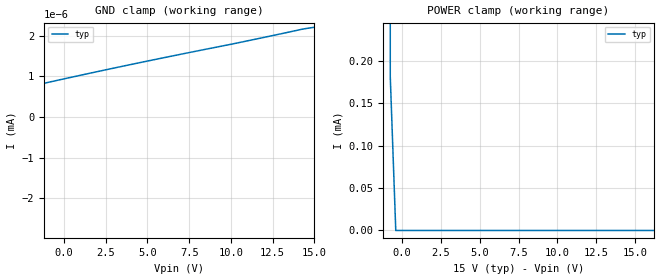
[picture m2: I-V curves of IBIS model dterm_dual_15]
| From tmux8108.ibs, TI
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| dterm_dual_15
[Model]   dterm_dual_15
Model_type   Terminator
|   typ   min   max
C_comp   1.008417e-11   NA   NA
[Voltage Range]   15   NA   NA
[Temperature Range]   27   NA   NA
[Power Clamp Reference]   15   NA   NA
[GND Clamp Reference]   0   NA   NA
[GND Clamp]
|   Voltage   I(typ)   I(min)   I(max)
-20V      -4.512A    NA         NA
-15.4V    -86.77nA   NA         NA
-15.05V   -296.1pA   NA         NA
-11.87V   -106.3pA   NA         NA
-9.394V   81.01pA    NA         NA
2.626V    1.175nA    NA         NA
15V       2.212nA    NA         NA
[POWER Clamp]
|   Voltage   I(typ)   I(min)   I(max)
-5V       1.488A     NA         NA
-1.111V   52.26mA    NA         NA
-757.6mV  181uA      NA         NA
-404mV    2.957nA    NA         NA
30V       -293pA     NA         NA
